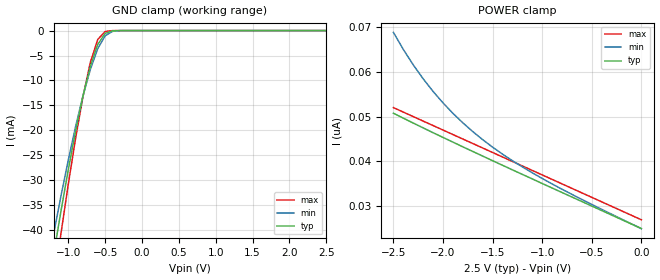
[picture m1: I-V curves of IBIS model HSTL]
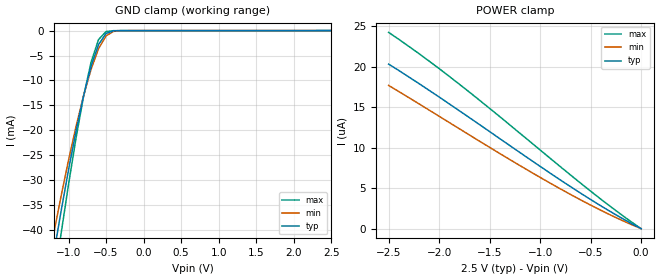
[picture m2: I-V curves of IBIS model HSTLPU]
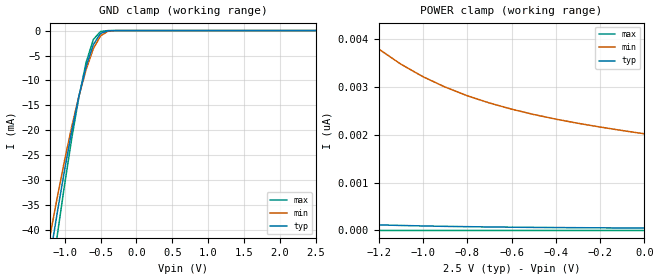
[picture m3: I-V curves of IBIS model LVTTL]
| IBIS file 72t1895.ibs created by s2ibis2 version 1.1
| North Carolina State University Electronics Research Laboratory  1995
[IBIS ver]   2.1
[File name]   72t1895.ibs
[File Rev]   1.0
[Date]   11/28/00
[Source]   Integrated Device Technology, Inc.
[Notes]   1. Temperatures: typ=25C, min=85C, max=-40C 2. Cemos11.5_2.5v
   process. 3. Ramp rates based on 50 ohm load.
[Copyright]   Copyright 1997, Integrated Device Technology, Inc.
|   Component idt72t1895z
[Component]   idt72t1895z
[Manufacturer]   Integrated Device Technology
[Package]
| variable   typ   min   max
R_pkg   0.75   0.60   0.90
L_pkg   8.10nH   8.30nH   9.90nH
C_pkg   0.53pF   0.46pF   0.60pF
| Note: The following pins list and their corresponding models based on
|   application.
|   The model_name is obvious and self-explanatory.
|   Please select the models accordingly.
|[Pin]  signal_name   model_name   R_pin   L_pin   C_pin
|   Dx(D0,...)   HSTL/EXHSTL/LVTTL
|   GND   GND
|   WENL   HSTL/EXHSTL/LVTTL
|   WCSL   HSTL/EXHSTL/LVTTL
|   WCLK   HSTL/EXHSTL/LVTTL
|   PRSL   HSTL/EXHSTL/LVTTL
|   MRSL   HSTL/EXHSTL/LVTTL
|   LDL   HSTL/EXHSTL/LVTTL
|   FWFTSI   HSTL/EXHSTL/LVTTL
|   FFL   FPAD_HSTL/FPAD_EXHSTL/FPAD_TTL
|   PAFL   FPAD_HSTL/FPAD_EXHSTL/FPAD_TTL
|   OW   LVTTL
|   FSEL0   LVTTL
|   HFL   FPAD_HSTL/FPAD_EXHSTL/FPAD_TTL
|   SHSTL   LVTTL
|   FSEL1   LVTTL
|   BEL   LVTTL
|   VDDQ   POWER
|   IP   LVTTL
|   BM   LVTTL
|   RHSTL   LVTTL
|   ASYRL   LVTTL
|   VCC   POWER
|   PAEL   FPAD_HSTL/FPAD_EXHSTL/FPAD_TTL
|   PFM   LVTTL
|   EFL   FPAD_HSTL/FPAD_EXHSTL/FPAD_TTL
|   ERENL   QPAD_HSTL/QPAD_EXHSTL/QPAD_TTL
|   MARK   HSTL/EXHSTL/LVTTL
|   RCLK   HSTL/EXHSTL/LVTTL
|   RENL   HSTL/EXHSTL/LVTTL
|   RTL   HSTL/EXHSTL/LVTTL
|   RCSL   HSTL/EXHSTL/LVTTL
|   OEL   HSTL/EXHSTL/LVTTL
|   Qx(Q0,...)   QPAD_HSTL/QPAD_EXHSTL/QPAD_TTL
|   ERCLK   QPAD_HSTL/QPAD_EXHSTL/QPAD_TTL
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[Pin]  signal_name   model_name   R_pin   L_pin   C_pin
1   HSTL   HSTL
2   EXHSTL   EXHSTL
3   LVTTL   LVTTL
4   VCC   POWER
5   GND   GND
6   FPAD_HSTL   FPAD_HSTL
7   FPAD_EXHSTL   FPAD_EXHSTL
8   FPAD_TTL   FPAD_TTL
9   QPAD_HSTL   QPAD_HSTL
10   QPAD_EXHSTL   QPAD_EXHSTL
11   QPAD_TTL   QPAD_TTL
12   HSTLPU   HSTLPU
13   EXHSTLPU   EXHSTLPU
14   LVTTLPU   LVTTLPU
| Models and submodels in the file (12): HSTL (Input), HSTLPU (Input), LVTTL (Input), LVTTLPU (Input), EXHSTL (Input), EXHSTLPU (Input), QPAD_HSTL (3-state), QPAD_TTL (3-state), QPAD_EXHSTL (3-state), FPAD_HSTL (3-state), FPAD_TTL (3-state), FPAD_EXHSTL (3-state)
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| FIN  FIN   dummy_model
| QIN  QIN   dummy_model
| QOE  QOE   dummy_model
| FOEL FOEL   dummy_model
|   Model HSTL
[Model]   HSTL
Model_type   Input
Vinl =  0.250V
Vinh =  1.250V
Vmeas =  0.750V
C_comp   3.00pF   NA   NA
[Temperature Range]   25.00   85.00   -40.00
[Voltage Range]   2.50V   2.30V   2.70V
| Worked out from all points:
|   GND clamp passes 1 mA (typ) near -0.52 V on its own axis
[GND_clamp]
| voltage   I(typ)   I(min)   I(max)
-2.5V     -171mA     -153mA     -195mA
-1.2V     -45.09mA   -40.91mA   -51.2mA
-1.1V     -36.28mA   -33.25mA   -40.8mA
-1V       -27.91mA   -25.98mA   -30.84mA
-900mV    -20.11mA   -19.21mA   -21.55mA
-800mV    -13.1mA    -13.07mA   -13.22mA
-700mV    -7.177mA   -7.773mA   -6.35mA
-600mV    -2.805mA   -3.616mA   -1.783mA
-500mV    -572uA     -1.059mA   -188uA
-400mV    -51.64uA   -157uA     -8.193uA
-300mV    -2.315uA   -13.07uA   -122nA
2.5V      25.05nA    27.16nA    25nA
[POWER_clamp]
| voltage   I(typ)   I(min)   I(max)
-2.5V     50.75nA    68.77nA    52nA
-2.4V     49.65nA    64.96nA    51nA
-2.3V     48.56nA    61.53nA    50nA
-2.2V     47.48nA    58.42nA    49nA
-2.1V     46.41nA    55.61nA    48nA
-1.9V     44.31nA    50.73nA    46nA
-1.8V     43.26nA    48.61nA    45nA
-1.6V     41.2nA     44.86nA    43nA
-1.3V     38.13nA    40.17nA    40nA
-1V       35.09nA    36.21nA    37nA
-600mV    31.07nA    31.53nA    33nA
0V        25.05nA    25.02nA    27nA
|   Model HSTLPU
[Model]   HSTLPU
Model_type   Input
Vinl =  0.250V
Vinh =  1.250V
Vmeas =  0.750V
C_comp   3.00pF   NA   NA
[Temperature Range]   25.00   85.00   -40.00
[Voltage Range]   2.50V   2.30V   2.70V
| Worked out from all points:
|   GND clamp passes 1 mA (typ) near -0.52 V on its own axis
[GND_clamp]
| voltage   I(typ)   I(min)   I(max)
-2.5V     -171mA     -153mA     -195mA
-1.2V     -45.09mA   -40.91mA   -51.21mA
-1.1V     -36.28mA   -33.25mA   -40.8mA
-1V       -27.91mA   -25.98mA   -30.84mA
-900mV    -20.12mA   -19.21mA   -21.55mA
-800mV    -13.11mA   -13.08mA   -13.22mA
-700mV    -7.179mA   -7.775mA   -6.354mA
-600mV    -2.808mA   -3.618mA   -1.788mA
-500mV    -576uA     -1.062mA   -195uA
-400mV    -56.63uA   -160uA     -15.52uA
-300mV    -7.47uA    -16.77uA   -7.499uA
2.5V      50.97pA    1.082uA    -1.591uA
[POWER_clamp]
| voltage   I(typ)   I(min)   I(max)
-2.5V     20.32uA    17.69uA    24.24uA
-2.2V     17.92uA    15.42uA    21.62uA
-1.8V     14.56uA    12.34uA    17.84uA
-900mV    6.85uA     5.617uA    8.684uA
-400mV    2.826uA    2.275uA    3.653uA
0V        50.97pA    2.018nA    220fA
|   Model LVTTL
[Model]   LVTTL
Model_type   Input
Vinl =  0.000V
Vinh =  2.500V
Vmeas =  1.250V
C_comp   3.00pF   NA   NA
[Temperature Range]   25.00   85.00   -40.00
[Voltage Range]   2.50V   2.30V   2.70V
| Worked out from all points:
|   GND clamp passes 1 mA (typ) near -0.52 V on its own axis
[GND_clamp]
| voltage   I(typ)   I(min)   I(max)
-2.5V     -171mA     -153mA     -195mA
-1.2V     -45.09mA   -40.91mA   -51.2mA
-1.1V     -36.28mA   -33.25mA   -40.8mA
-1V       -27.91mA   -25.98mA   -30.84mA
-900mV    -20.11mA   -19.21mA   -21.55mA
-800mV    -13.1mA    -13.07mA   -13.22mA
-700mV    -7.177mA   -7.773mA   -6.35mA
-600mV    -2.805mA   -3.616mA   -1.783mA
-500mV    -571uA     -1.059mA   -188uA
-400mV    -51.63uA   -157uA     -8.189uA
-300mV    -2.312uA   -13.07uA   -119nA
2.5V      50.98pA    2.159nA    204fA
[POWER_clamp]
| voltage   I(typ)   I(min)   I(max)
-2.5V     750pA      20.77nA    2.711pA
-2.3V     558pA      15.53nA    2.052pA
-2V       355pA      10.06nA    1.341pA
-1.7V     228pA      6.656nA    893fA
-1.3V     132pA      4.17nA     553fA
-1.2V     117pA      3.787nA    493fA
-1.1V     105pA      3.471nA    451fA
-1V       94.88pA    3.209nA    410fA
-800mV    79.45pA    2.812nA    350fA
-500mV    64.69pA    2.421nA    286fA
-300mV    58.18pA    2.237nA    256fA
0V        50.98pA    2.018nA    221fA
